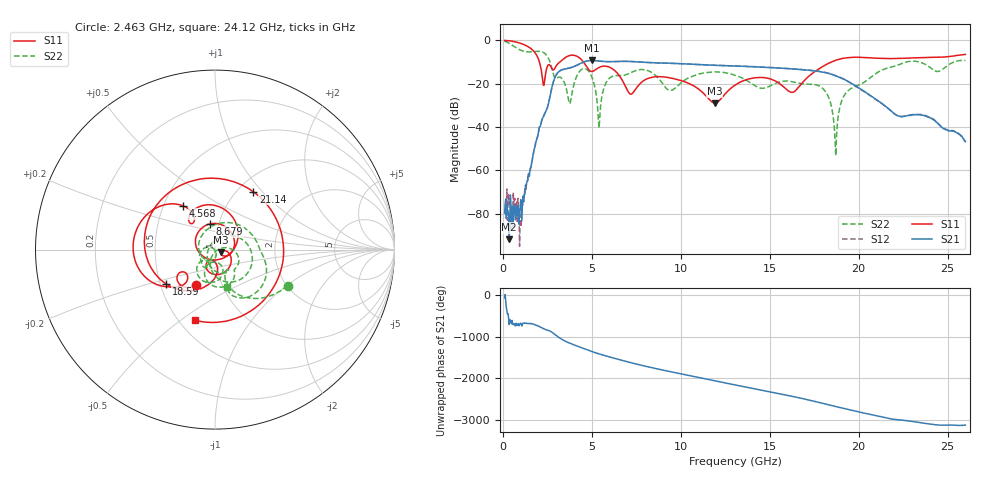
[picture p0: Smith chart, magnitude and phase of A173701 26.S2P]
!  2-Port S-parameters saved by WinCal
! VAR MeasName=S-Parameters (CALIBRATED_DATA) read from VNA (N5245A)
! VAR MeasDate=2017-6-7 10:30:06
! VAR NAME=A173701 26
! VAR FILENAME=A173701 26.S2P
! VAR DATE=2017-6-7 10:30:06
! VAR PHYS_PORTS=1,2
# Hz S DB R 50
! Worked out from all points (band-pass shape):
!   801 points, 100 MHz to 26 GHz, reference 50 ohm
!   highest |S21| = -9.25 dB at 5.021 GHz (marker M1); lowest = -91.8 dB at 359 MHz (marker M2)
!   |S21| within 3 dB of the highest: 3.936 GHz to 14.29 GHz (10.35 GHz wide, 114 % of centre)
!   lowest |S11| = -28.9 dB at 11.92 GHz (marker M3), VSWR 1.07, Z = 53.3 - j1.56 ohm
!   |S11| at or under -10 dB: 2.057 GHz to 3.199 GHz (1.142 GHz wide, 43.4 % of centre); 4.533 GHz to 18.46 GHz (13.93 GHz wide, 121 % of centre)
!   |S22| runs from -53.1 to -0.3 dB; largest |S21 - S12| = 0.0039
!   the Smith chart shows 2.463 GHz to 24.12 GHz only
!   S11 on the Smith chart (normalised r, x): 2.463 GHz: 0.75, -0.32; 4.568 GHz: 0.63, +0.34; 8.679 GHz: 0.91, +0.27; 18.59 GHz: 0.54, -0.23; 21.14 GHz: 1.18, +0.89; 24.12 GHz: 0.60, -0.57
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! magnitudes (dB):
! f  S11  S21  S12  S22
! 100 MHz  0.0  -79.7  -79.8  -0.3
! 359 MHz  -0.2  -91.8  -75.8  -1.3
! 1.039 GHz  -1.5  -78.7  -80.4  -4.6
! 2.463 GHz  -12.9  -31.9  -31.9  -6.9
! 3.758 GHz  -7.0  -12.7  -12.7  -29.2
! 4.438 GHz  -9.1  -10.3  -10.4  -13.3
! 4.568 GHz  -10.4  -9.9  -9.9  -13.0
! 5.021 GHz  -14.3  -9.2  -9.3  -17.3
! 5.41 GHz  -12.5  -9.5  -9.5  -40.5
! 6.089 GHz  -12.7  -9.8  -9.8  -16.9
! 7.19 GHz  -24.8  -9.7  -9.7  -14.9
! 8.679 GHz  -16.7  -10.4  -10.4  -16.9
! 8.744 GHz  -16.7  -10.4  -10.4  -17.5
! 11.92 GHz  -28.9  -11.5  -11.5  -14.5
! 13.05 GHz  -20.6  -11.8  -11.8  -16.1
! 17.39 GHz  -15.3  -14.0  -13.9  -20.3
! 18.23 GHz  -10.9  -15.1  -15.0  -24.8
! 18.59 GHz  -9.6  -16.0  -15.9  -36.4
! 21.14 GHz  -8.3  -28.2  -28.3  -14.4
! 21.69 GHz  -8.4  -31.6  -31.6  -12.6
! 24.12 GHz  -7.8  -36.2  -36.0  -13.2
! 26 GHz  -6.5  -46.7  -46.7  -9.3
